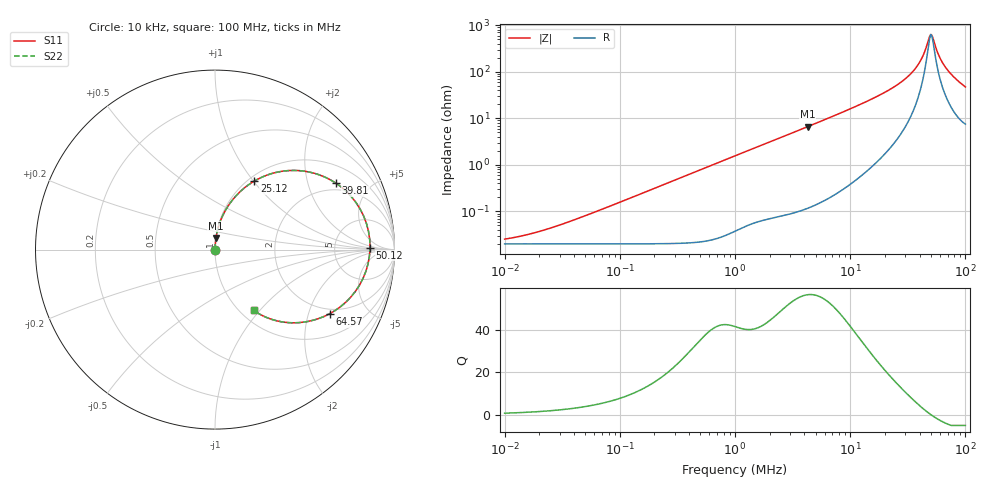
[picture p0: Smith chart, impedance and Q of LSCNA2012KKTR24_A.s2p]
! LSCNA2012KKTR24_A  S-PARAMETER MODEL  ( Standard Model )
! Model Generated by TAIYO YUDEN Corporation (http://www.ty-top.com)
! Version 2.0
! TAIYO YUDEN Control No. 171005
! Copyright(c) 2016 TAIYO YUDEN CO.,LTD. All Rights Reserved.
! Product Description (link to TY-COMPAS)
! https://ds.yuden.co.jp/TYCOMPAS/or/detail?pn=LSCNA2012KKTR24MA&u=M
! Products Name : Inductors
! Characteristics :
!  Inductance : 0.24 [uH] , SRF(min) : - [Hz] , DC Resistance(max) : 25 [mOhm]
!  Rated Current : Saturation  6.2 [A] (dL = 30 [%]), Temp Rise  4.0 [A] (dT = 40 [degC])
!  Case Size : 2.0 x 1.25 / 0.079 x 0.049 [mm/inch] , Thickness : 1.0 / 0.039 [mm/inch]
!  (Conditions: Temperature = 25 [degC] , DC Bias Current = 0 [A])
! External Node Assignments :
!  1  o---GGG---o  2
! GND o---------o GND
! Frequency Range : 10kHz  -  100MHz  [ 402 STEP ]
# MHz S RI R 50
! Freq[MHz].  S11 Real  S11 Imag  S21 Real  S21 Imag  S12 Real  S12 Imag  S22 Real  S22 Imag
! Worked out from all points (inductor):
!   401 points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, 10 kHz to 100 MHz, reference 50 ohm
!   read as one part in series: L = 248 nH near 38.91 kHz
!   highest Q = 56.7 at 4.266 MHz (marker M1), where L = 246 nH
!   self-resonance near 50.42 MHz
!   S11 on the Smith chart (normalised r, x): 10 kHz: 1.00, +0.00; 25.12 MHz: 1.07, +1.01; 39.81 MHz: 1.68, +3.04; 50.12 MHz: 14, +1; 64.57 MHz: 1.80, -2.77; 100 MHz: 1.15, -0.93
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0.01  0.0002 0.000156  0.9998 -0.000156  0.9998 -0.000156  0.0002 0.000156
0.019953  0.0002 0.000311  0.9998 -0.000311  0.9998 -0.000311  0.0002 0.000311
0.046774  0.000201 0.000729  0.9998 -0.000729  0.9998 -0.000729  0.000201 0.000729
0.218776  0.000214 0.00341  0.9998 -0.00341  0.9998 -0.00341  0.000214 0.00341
1  0.000619 0.0156  0.9994 -0.0156  0.9994 -0.0156  0.000619 0.0156
4.265795  0.00548 0.0655  0.9945 -0.0655  0.9945 -0.0655  0.00548 0.0655
4.677351  0.00647 0.0719  0.9935 -0.0719  0.9935 -0.0719  0.00647 0.0719
12.58925  0.0457 0.1949  0.9543 -0.1949  0.9543 -0.1949  0.0457 0.1949
21.87762  0.157 0.338  0.843 -0.338  0.843 -0.338  0.157 0.338
25.11886  0.2197 0.3822  0.7803 -0.3822  0.7803 -0.3822  0.2197 0.3822
33.11311  0.4412 0.4412  0.5588 -0.4412  0.5588 -0.4412  0.4412 0.4412
39.81072  0.6739 0.3702  0.3261 -0.3702  0.3261 -0.3702  0.6739 0.3702
42.65795  0.7609 0.2936  0.2391 -0.2936  0.2391 -0.2936  0.7609 0.2936
45.70882  0.8286 0.1861  0.1714 -0.1861  0.1714 -0.1861  0.8286 0.1861
47.86301  0.8554 0.1011  0.1446 -0.1011  0.1446 -0.1011  0.8554 0.1011
50.11872  0.8638 0.0109  0.1362 -0.0109  0.1362 -0.0109  0.8638 0.0109
52.48075  0.8528 -0.0787  0.1472 0.0787  0.1472 0.0787  0.8528 -0.0787
57.54399  0.7809 -0.2345  0.2191 0.2345  0.2191 0.2345  0.7809 -0.2345
64.56542  0.639 -0.3573  0.361 0.3573  0.361 0.3573  0.639 -0.3573
77.62471  0.4147 -0.4072  0.5853 0.4072  0.5853 0.4072  0.4147 -0.4072
89.12509  0.2899 -0.3794  0.7101 0.3794  0.7101 0.3794  0.2899 -0.3794
100  0.2163 -0.339  0.7837 0.339  0.7837 0.339  0.2163 -0.339
